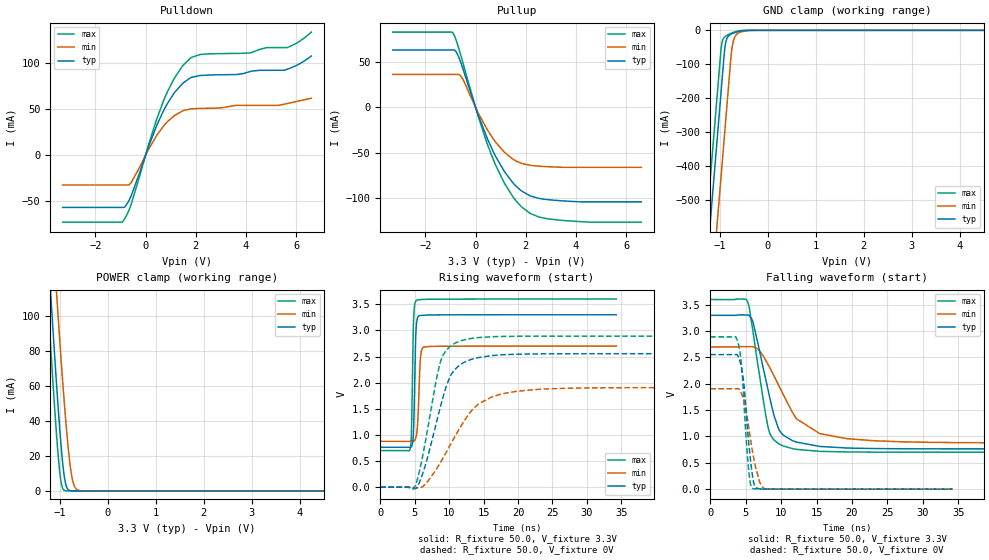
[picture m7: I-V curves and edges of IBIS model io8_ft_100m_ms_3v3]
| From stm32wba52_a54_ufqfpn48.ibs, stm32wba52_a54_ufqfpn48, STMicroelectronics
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[Model]   io8_ft_100m_ms_3v3
Model_type I/O
Polarity   Non-Inverting
Enable   Active-Low
| CAP_THRESHOLD on pad IOFT is "UDTCAPC" :
| Rising=30.0% of vddiom   Falling=70.0% of vddiom
| C_comp min and max val. don't necessarily correlate with the min and max pvt
| but are the smallest and greatest pad capacitance found.
| var   typ   min   max
C_comp   2.69682pF  2.55496pF  2.73061pF
|C_comp_pullup   1.75285pF  1.65246pF  1.79141pF
|C_comp_pulldown   943.96933fF  902.50346fF  939.20299fF
Vinl = 1.35V
Vinh = 1.8V
Vmeas = 1.65V   | Reference voltage for timing measurements
Cref  = 50.0pF   | Timing specification test load capacitance value
Rref  = 1.0MOhm   | Timing specification test load resistance value
Vref  = 1.815V   | Timing specification test load voltage
[Model Spec]
| TIME_THRESHOLD on pin ZIV11 is "CMOS" :
| Rising=50.0% of vdd   Falling=50.0% of vdd
Vinl 1.29050V 1.08150V 1.39050V
Vinh 1.79850V 1.49250V 1.94450V
| variable   typ   min   max
[Temperature Range] 25.0 140.0 -40.0
| variable   typ   min   max
[Voltage Range] 3.3V 2.7V 3.6V
| variable   typ   min   max
[POWER Clamp Reference] 3.3V 2.7V 3.6V
| variable   typ   min   max
[GND Clamp Reference] 0V 0V 0V
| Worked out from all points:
|   slope of the pulldown table from 0 to 0.495 V, typ, clamps not added: 14 ohm
|   slope of the pullup table from 0 to 0.495 V, typ, clamps not added: 13.8 ohm
|   GND clamp passes 1 mA (typ) near -0.51 V on its own axis
|   POWER clamp passes 1 mA (typ) near -0.83 V on its own axis
|   rising waveform, R_fixture 50.0, V_fixture 3.3V: 20-80 % time 257ps typ, 336ps min, 230ps max; typ from 0.764 V to 3.3 V
|   falling waveform, R_fixture 50.0, V_fixture 3.3V: 20-80 % time 2.64ns typ, 4.97ns min, 2ns max; typ from 3.3 V to 0.764 V
|   rising waveform, R_fixture 50.0, V_fixture 0V: 20-80 % time 3.17ns typ, 5.37ns min, 2.44ns max; typ from 0 V to 2.55 V
|   falling waveform, R_fixture 50.0, V_fixture 0V: 20-80 % time 1.01ns typ, 1.46ns min, 849ps max; typ from 2.55 V to 0 V
[POWER Clamp]
-3.3V     1.123A     1.139A     1.091A
-1.36V    189.2mA    238.8mA    158.1mA
-1.25V    139mA      190.3mA    108.1mA
-1.18V    107.9mA    159.9mA    77.22mA
-1.06V    57.23mA    109.3mA    28.68mA
-980mV    27.6mA     77.28mA    5.935mA
-900mV    6.895mA    47.74mA    242.8uA
-820mV    594.6uA    22.85mA    5.912uA
-760mV    69.41uA    9.714mA    358.6nA
-700mV    7.83uA     2.919mA    21.86nA
-630mV    611.5nA    529.9uA    954.5pA
6.6V      0A         0A         0A
[GND Clamp]
-3.3V     -4.134A    -4.382A    -4.006A
-1.59V    -1.227A    -1.475A    -1.099A
-1.25V    -648.9mA   -896.7mA   -520.9mA
-980mV    -189.9mA   -437.7mA   -61.92mA
-970mV    -172.9mA   -420.7mA   -48.45mA
-910mV    -70.86mA   -318.7mA   -21.03mA
-880mV    -37.23mA   -267.7mA   -17.31mA
-750mV    -9.908mA   -55.25mA   -7.768mA
-710mV    -7.626mA   -27.41mA   -5.608mA
-650mV    -4.885mA   -11.6mA    -3.058mA
-360mV    -31.22uA   -443.6uA   -1.188uA
6.6V      2.31nA     2.655uA    974.6pA
| variable   typ   min   max
[Pullup Reference] 3.3V 2.7V 3.6V
| variable   typ   min   max
[Pulldown Reference] 0V 0V 0V
[Pullup]
-3.3V     63.23mA    36.27mA    82.93mA
-900mV    63.23mA    36.27mA    81.84mA
-750mV    60mA       36.27mA    72.08mA
-540mV    45.51mA    32.55mA    52.64mA
120mV     -9.566mA   -6.929mA   -11.25mA
710mV     -49.08mA   -34.92mA   -57.81mA
1.14V     -70.33mA   -49.14mA   -83.06mA
1.48V     -82.86mA   -56.83mA   -98.19mA
1.83V     -91.98mA   -61.62mA   -109.5mA
2.17V     -97.42mA   -63.75mA   -116.7mA
2.85V     -101.5mA   -65.23mA   -122.5mA
6.6V      -104mA     -65.97mA   -126.4mA
[Pulldown]
-3.3V     -56.7mA    -32.4mA    -72.73mA
-890mV    -56.7mA    -32.4mA    -71.32mA
-570mV    -43.94mA   -29.54mA   -52.99mA
120mV     9.474mA    6.407mA    11.48mA
700mV     47.33mA    30.97mA    57.88mA
1.14V     67.41mA    42.74mA    83.2mA
1.78V     83.75mA    50.04mA    105.1mA
2.17V     86.37mA    50.65mA    109.1mA
4.16V     90.61mA    53.89mA    110.8mA
4.82V     92.03mA    53.89mA    116.6mA
5.63V     93.04mA    55.89mA    116.6mA
6.6V      107.5mA    61.71mA    133.4mA
[Ramp]
dV/dt_r 1.53258V/3.14461ns 1.14345V/5.34827ns 1.73412V/2.42916ns
dV/dt_f 1.52157V/2.56911ns 1.09312V/4.46735ns 1.73923V/2.00141ns
R_load = 50.0
| Removed startup time: 0s 0s 0s  .
| Removed end time: 34.25ns.
[Rising Waveform]
R_fixture   = 50.0
V_fixture   = 3.3V
V_fixture_min = 2.7V
V_fixture_max = 3.6V
0s        764mV      878.1mV    701.3mV
4.35ns    761.3mV    877.9mV    739.2mV
4.55ns    783.2mV    876.8mV    1.181V
4.85ns    1.168V     880.2mV    3.252V
5.1ns     2.664V     923.1mV    3.548V
5.25ns    3.119V     996.4mV    3.575V
5.45ns    3.253V     1.282V     3.584V
5.85ns    3.286V     2.494V     3.589V
6.3ns     3.291V     2.68V      3.594V
34.25ns   3.3V       2.7V       3.6V
| Removed startup time: 0s 0s 0s  .
| Removed end time: 189.25ns.
[Falling Waveform]
R_fixture   = 50.0
V_fixture   = 3.3V
V_fixture_min = 2.7V
V_fixture_max = 3.6V
0s        3.3V       2.7V       3.6V
5.2ns     3.307V     2.706V     3.575V
6.05ns    3.162V     2.702V     2.974V
7.5ns     2.279V     2.524V     1.677V
8.35ns    1.764V     2.319V     1.081V
9.7ns     1.125V     1.957V     858.6mV
12.15ns   893.9mV    1.337V     755.1mV
15.45ns   811.1mV    1.055V     718mV
27.05ns   766.8mV    899.1mV    701.9mV
189.3ns   764mV      878.1mV    701.3mV
| Removed startup time: 0s 0s 0s  .
| Removed end time: 99.2ns.
[Rising Waveform]
R_fixture   = 50.0
V_fixture   = 0V
V_fixture_min = 0V
V_fixture_max = 0V
0s        20.8nV     574.2nV    32.98nV
4.95ns    -20.9mV    -6.11mV    -8.404mV
6.45ns    377.9mV    48.21mV    799.6mV
7.95ns    1.13V      303.2mV    1.925V
8.8ns     1.573V     488.2mV    2.425V
10.4ns    2.178V     866.8mV    2.72V
12.65ns   2.418V     1.36V      2.833V
16.2ns    2.518V     1.728V     2.879V
24.3ns    2.552V     1.882V     2.89V
99.2ns    2.554V     1.906V     2.89V
| Removed startup time: 0s 0s 0s  .
| Removed end time: 34.2ns.
[Falling Waveform]
R_fixture   = 50.0
V_fixture   = 0V
V_fixture_min = 0V
V_fixture_max = 0V
0s        2.554V     1.906V     2.89V
3.55ns    2.554V     1.906V     2.894V
4ns       2.499V     1.907V     2.741V
4.35ns    2.339V     1.828V     2.421V
4.7ns     2.052V     1.7V       1.764V
5.4ns     919.6mV    1.199V     388.7mV
5.95ns    261.7mV    723.2mV    16.22mV
7ns       4.094mV    122.1mV    2.163mV
7.7ns     2.289mV    11mV       1.504mV
34.2ns    5.238uV    32.47uV    1.269uV
